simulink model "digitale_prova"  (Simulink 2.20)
settings: Solver=VariableStepDiscrete  StartTime=0.0  StopTime=10.0  RelTol=1e-3  AbsTol=1e-6

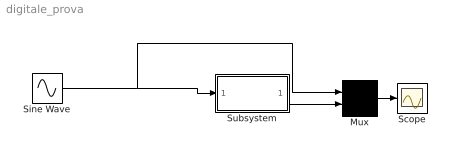
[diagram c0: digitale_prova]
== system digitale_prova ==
  Mux : Mux  Inputs=2
  Scope : Scope
  Sine Wave : Sin  Amplitude=1  Frequency=1  Phase=0  SampleTime=0
  Subsystem : Subsystem  mask(inserisci i parametri){Kp=3}
      mask prompts: Kp "guadagno"
      mask init:
      | Ko=Kp*2;
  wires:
  Mux/1 -> Scope/1
  Subsystem/1(Out1) -> Mux/2
  Sine Wave/1 -> Subsystem/1(In1), Mux/1

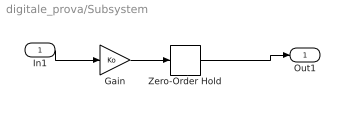
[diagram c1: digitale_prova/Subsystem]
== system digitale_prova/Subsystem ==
  In1 : Inport  Port=1  PortWidth=-1  SampleTime=-1
  Gain : Gain  Gain=Ko
  Zero-Order Hold : ZeroOrderHold  SampleTime=1
  Out1 : Outport  Port=1
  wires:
  Zero-Order Hold/1 -> Out1/1
  In1/1 -> Gain/1
  Gain/1 -> Zero-Order Hold/1
